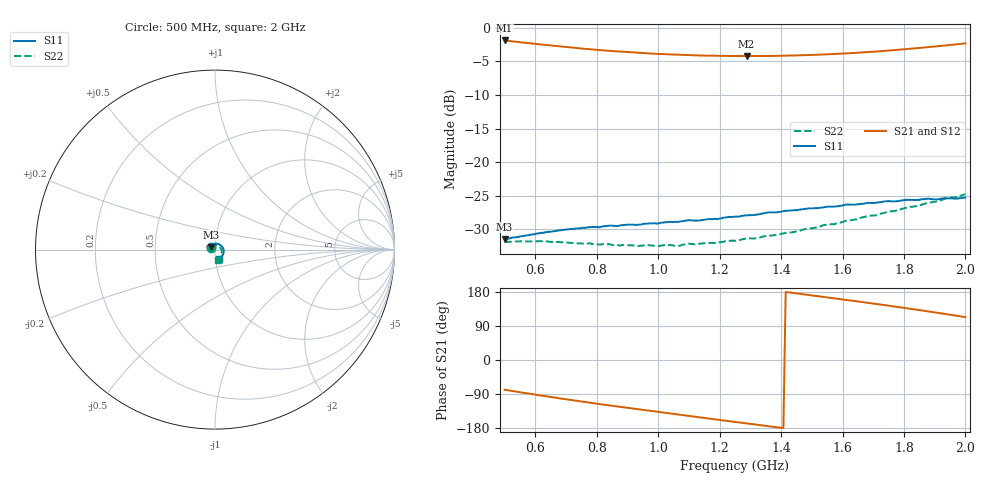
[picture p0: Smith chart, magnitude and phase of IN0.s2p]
!Agilent Technologies,E8363B,SG43030131,A.07.50.48
!Agilent E8363B: A.07.50.48
!Date: Thursday, October 16, 2025 22:14:01
!Correction: S11(Full 2 Port(1,2))
!S21(Full 2 Port(1,2))
!S12(Full 2 Port(1,2))
!S22(Full 2 Port(1,2))
!S2P File: Measurements: S11, S21, S12, S22:
# Hz S  dB  R 50
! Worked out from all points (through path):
!   201 points, 500 MHz to 2 GHz, reference 50 ohm
!   highest |S21| = -1.91 dB at 500 MHz (marker M1); lowest = -4.2 dB at 1.288 GHz (marker M2)
!   group delay of S21, straight-line fit = 302 ps
!   lowest |S11| = -31.4 dB at 500 MHz (marker M3), VSWR 1.06, Z = 47.8 + j1.35 ohm
!   |S11| at or under -10 dB: start of sweep to end of sweep
!   |S22| runs from -32.5 to -24.8 dB; largest |S21 - S12| = 0.0016
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5e8  -31.42 148.1  -1.91 -78.6  -1.91 -78.5  -31.87 156.5
5.6e8  -30.98 134.4  -2.22 -86.4  -2.23 -86.4  -31.78 145.8
6.275e8  -30.50 120.4  -2.55 -94.9  -2.56 -94.9  -31.77 133.9
7.55e8  -29.76 99.5  -3.12 -110.1  -3.13 -110.1  -32.12 115.1
8.675e8  -29.50 83.0  -3.54 -122.8  -3.54 -122.9  -32.34 99.7
1.0025e9  -29.08 65.9  -3.91 -137.5  -3.93 -137.4  -32.49 82.2
1.025e9  -28.93 62.9  -3.96 -139.9  -3.97 -139.9  -32.30 79.5
1.07e9  -28.84 57.7  -4.05 -144.6  -4.06 -144.6  -32.44 73.7
1.1e9  -28.62 54.3  -4.09 -147.8  -4.10 -147.7  -32.14 69.2
1.1225e9  -28.67 51.9  -4.13 -150.1  -4.13 -150.1  -32.28 66.7
1.16e9  -28.50 47.4  -4.17 -154.0  -4.18 -154.0  -31.97 61.8
1.1825e9  -28.43 44.2  -4.20 -156.4  -4.20 -156.4  -32.03 58.8
1.25e9  -28.09 37.1  -4.22 -163.3  -4.24 -163.4  -31.69 49.2
1.2875e9  -27.92 33.1  -4.24 -167.2  -4.25 -167.2  -31.30 44.3
1.325e9  -27.78 28.7  -4.23 -171.2  -4.24 -171.1  -31.29 39.5
1.355e9  -27.50 25.7  -4.22 -174.2  -4.23 -174.2  -30.95 34.3
1.505e9  -26.86 9.2  -4.05 170.1  -4.07 170.1  -29.81 11.8
1.6325e9  -26.32 -6.5  -3.78 156.4  -3.78 156.4  -28.61 -8.7
1.7525e9  -25.81 -23.0  -3.40 143.1  -3.41 143.1  -27.34 -28.9
1.88e9  -25.44 -43.5  -2.89 128.2  -2.90 128.2  -26.02 -52.0
1.94e9  -25.37 -54.8  -2.63 120.8  -2.63 120.8  -25.37 -63.8
2e9  -25.27 -67.5  -2.34 113.2  -2.35 113.2  -24.79 -75.8
